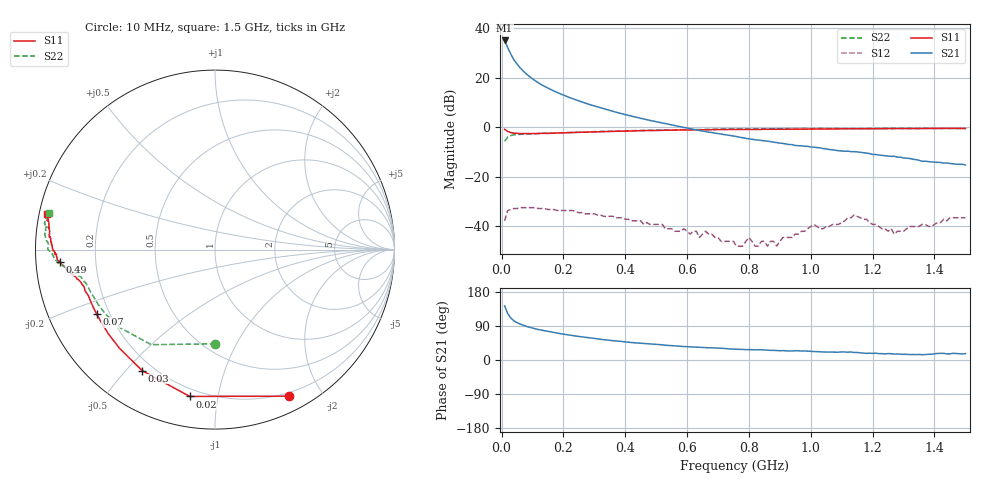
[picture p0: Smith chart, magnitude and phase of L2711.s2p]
!Date: Fri Aug 27 15:04:00 1999
!  POLYFET RF DEVICES
!  L2711
!  7.5Vdc		400ma
# MHZ  S  MA  R  50.0000
! SCATTERING PARAMETERS :
! Freq=MHz Mag[s11] Ang[s11] Mag[s21] Ang[s21] Mag[s12] Ang[s12] Mag[s22] Ang[s22]
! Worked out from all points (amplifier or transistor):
!   150 points, 10 MHz to 1.5 GHz, reference 50 ohm
!   highest |S21| = 35.1 dB at 10 MHz (marker M1)
!   |S21| within 3 dB of that: start of sweep to 20.4 MHz
!   unconditionally stable (mu >= 1): 453.7 MHz to end of sweep
!   at 260 MHz: K = 0.46, MSG = 22.4 dB, |S12| = -34.4 dB
!   at 760 MHz: K = 3.87, MAG = 13.3 dB, |S12| = -48.0 dB
!   at 1.5 GHz: K = 2.30, MAG = 4.3 dB, |S12| = -36.5 dB
!   S11 on the Smith chart (normalised r, x): 10 MHz: 0.16, -1.61; 20 MHz: 0.16, -0.83; 30 MHz: 0.16, -0.56; 70 MHz: 0.15, -0.25; 490 MHz: 0.07, -0.04; 1.5 GHz: 0.02, +0.10
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10  0.915 -63.2  57.03 142.9  0.013 51.9  0.525 -89.7
20  0.83 -99.8  40.87 122.5  0.021 32.5  0.638 -123.9
30  0.787 -121.0  30.18 110.9  0.022 20.8  0.684 -140.4
40  0.765 -134.1  23.33 103.4  0.023 15.2  0.708 -149.6
50  0.757 -141.9  19.15 98.8  0.023 10.4  0.719 -154.7
60  0.752 -147.4  16.06 94.9  0.024 5.9  0.724 -158.2
70  0.751 -151.5  13.79 91.7  0.024 2.8  0.732 -160.9
80  0.75 -154.6  12.1 88.9  0.024 2.8  0.735 -162.6
100  0.75 -159.0  9.593 84.3  0.024 -3.2  0.742 -165.3
130  0.76 -162.6  7.234 78.8  0.023 -7.7  0.758 -167.5
180  0.769 -166.4  5.081 71.1  0.021 -12.0  0.775 -169.1
260  0.798 -169.4  3.265 60.9  0.019 -18.4  0.806 -171.2
360  0.83 -172.2  2.112 50.9  0.016 -25.5  0.842 -172.9
490  0.866 -175.4  1.346 41.9  0.011 -25.6  0.878 -175.5
510  0.872 -175.9  1.267 40.4  0.011 -26.0  0.883 -176.0
760  0.911 178.3  0.655 28.3  0.004 16.3  0.929 179.0
800  0.911 178.0  0.589 27.5  0.006 40.1  0.929 178.1
890  0.918 176.0  0.494 24.9  0.004 57.9  0.941 177.0
1010  0.926 174.6  0.4 22.3  0.011 74.0  0.951 174.3
1140  0.936 172.3  0.324 19.9  0.017 67.5  0.946 172.3
1260  0.946 169.7  0.26 16.6  0.009 57.1  0.961 170.8
1500  0.954 168.1  0.175 16.8  0.015 85.0  0.947 167.4
